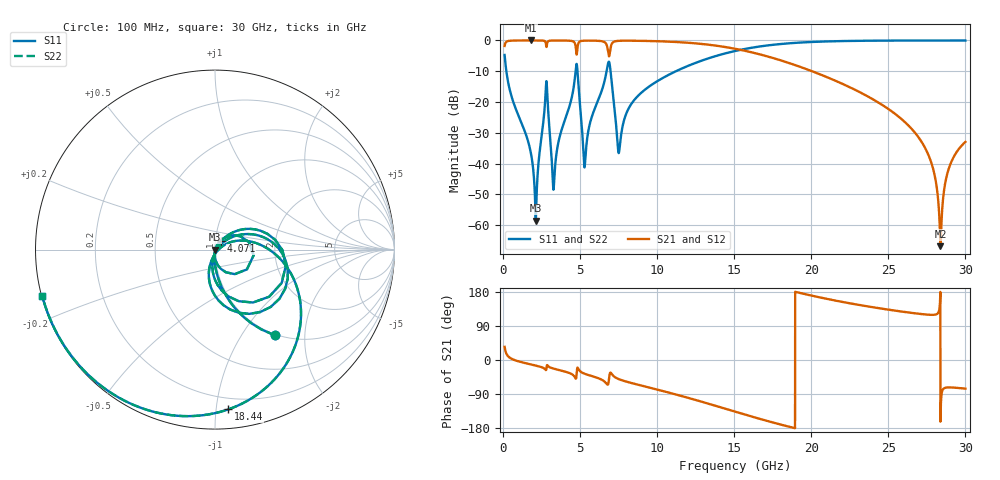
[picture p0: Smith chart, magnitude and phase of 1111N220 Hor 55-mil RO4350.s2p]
# GHz S MA R 50
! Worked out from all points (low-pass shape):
!   3201 points, 100 MHz to 30 GHz, reference 50 ohm
!   highest |S21| = -0.01 dB at 1.801 GHz (marker M1); lowest = -66.9 dB at 28.38 GHz (marker M2)
!   |S21| within 3 dB of the highest: start of sweep to 4.735 GHz; 6.954 GHz to 15.36 GHz (8.404 GHz wide, 75.3 % of centre)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
!   lowest |S11| = -58.6 dB at 2.118 GHz (marker M3), VSWR 1.00, Z = 50.1 - j0.0526 ohm
!   |S11| at or under -10 dB: 212.8 MHz to 4.703 GHz (4.491 GHz wide, 183 % of centre); 4.828 GHz to 6.718 GHz (1.889 GHz wide, 32.7 % of centre); 6.975 GHz to 11.22 GHz (4.245 GHz wide, 46.7 % of centre)
!   |S22| runs from -58.6 to 0.0 dB; largest |S21 - S12| = 0
!   S11 on the Smith chart (normalised r, x): 100 MHz: 0.98, -1.41; 4.071 GHz: 1.06, +0.10; 18.44 GHz: 0.12, -1.08; 30 GHz: 0.00, -0.13
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0.1  0.5806 -55.2  0.8139 34.8  0.8139 34.8  0.5806 -55.2
1.800563  0.01498 -98.4  0.9988 -11.7  0.9988 -11.7  0.01498 -98.4
2.11825  0.001181 -26.4  0.9986 -14.7  0.9986 -14.7  0.001181 -26.4
2.772312  0.1598 27.6  0.898 -26.7  0.898 -26.7  0.1598 27.6
3.286219  0.003994 3.0  0.996 -22.8  0.996 -22.8  0.003994 3.0
4.071094  0.05614 55.1  0.9943 -31.2  0.9943 -31.2  0.05614 55.1
4.753188  0.4047 -12.6  0.6343 -45.1  0.6343 -45.1  0.4047 -12.6
5.089563  0.04568 -100.8  0.9817 -32.3  0.9817 -32.3  0.04568 -100.8
5.341844  0.01243 15.5  0.9918 -37.0  0.9918 -37.0  0.01243 15.5
6.8275  0.4358 -21.5  0.6291 -62.7  0.6291 -62.7  0.4358 -21.5
7.528281  0.01541 -24.0  0.9854 -50.8  0.9854 -50.8  0.01541 -24.0
8.266438  0.08839 26.2  0.9894 -60.0  0.9894 -60.0  0.08839 26.2
10.06978  0.2225 10.2  0.9698 -78.7  0.9698 -78.7  0.2225 10.2
15.05  0.6728 -46.7  0.7323 -136.2  0.7323 -136.2  0.6728 -46.7
18.44178  0.8933 -85.3  0.4388 -174.8  0.4388 -174.8  0.8933 -85.3
20.03956  0.9441 -100.7  0.3166 169.7  0.3166 169.7  0.9441 -100.7
25.01978  0.9937 -137.9  0.07638 132.8  0.07638 132.8  0.9937 -137.9
27.49588  0.9966 -152.2  0.01578 119.8  0.01578 119.8  0.9966 -152.2
28.00978  0.9967 -154.9  0.006361 119.5  0.006361 119.5  0.9967 -154.9
28.38353  0.9967 -156.8  0.0004541 -162.7  0.0004541 -162.7  0.9967 -156.8
28.92547  0.9967 -159.6  0.008322 -72.3  0.008322 -72.3  0.9967 -159.6
30  0.9965 -164.8  0.02247 -75.6  0.02247 -75.6  0.9965 -164.8
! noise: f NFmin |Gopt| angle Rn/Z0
0.1  0.0007042  0.7495  2.43  0.0005659
3.417  0.01377  0.6005  23.52  0.006103
6.743  0.1369  0.9083  45.35  0.2794
10.06  0.02799  0.4959  62.43  0.007285
13.39  0.0377  0.5245  76.94  0.009053
16.7  0.05723  0.625  92.55  0.01443
20.03  0.09916  0.7569  110.6  0.02783
23.35  0.2139  0.8792  129.6  0.07064
26.67  0.8514  0.968  148  0.4612
30  1.252  0.9776  164.7  0.2294
